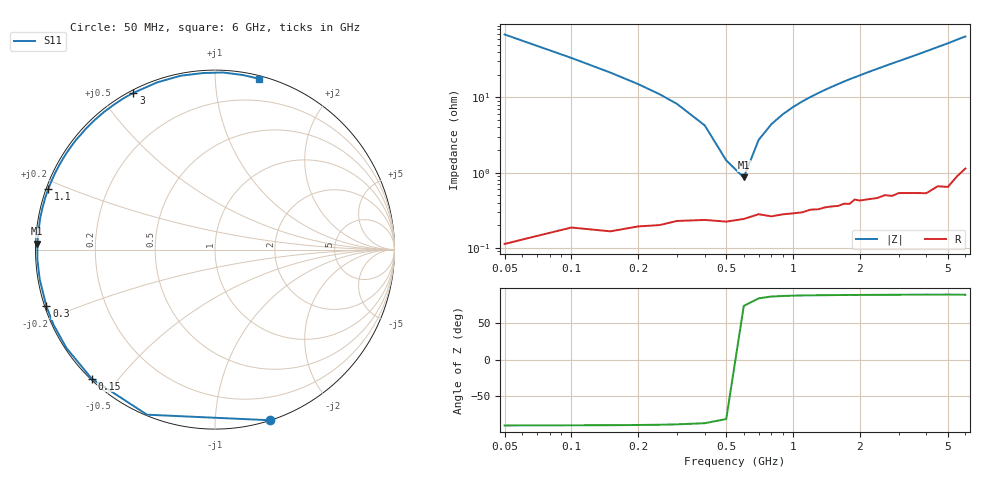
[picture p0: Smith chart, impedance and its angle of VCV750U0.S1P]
! Infineon Technologies  Discrete & RF Semiconductors
! BBY 56-03
! Si Tuning Diode in SOD323
! VR = 0.75 V
! S-Parameters:  June  1999
# GHz  S  MA  R  50
!  f  S11
! GHz  MAG  ANG
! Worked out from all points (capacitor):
!   34 points, 50 MHz to 6 GHz, reference 50 ohm
!   read as one part to ground: C = 46.1 pF near 50 MHz
!   lowest |Z| = 864 mohm at 600 MHz (marker M1)
!   series resonance near 563.5 MHz, so ESL is about 1.7 nH
!   S11 on the Smith chart (normalised r, x): 50 MHz: 0.00, -1.37; 150 MHz: 0.00, -0.43; 300 MHz: 0.00, -0.16; 1.1 GHz: 0.01, +0.18; 3 GHz: 0.01, +0.61; 6 GHz: 0.02, +1.29
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0.05  0.9984 -72.2
0.1  0.9949 -112.4
0.15  0.9944 -133.7
0.2  0.9929 -146.5
0.25  0.9923 -155.1
0.3  0.9911 -161.4
0.4  0.9907 -170.3
0.5  0.9911 -176.7
0.6  0.9903 178.1
0.7  0.9889 173.8
0.8  0.9896 169.9
1  0.9888 163.1
1.1  0.9885 160.0
1.3  0.9877 154.3
1.6  0.9868 146.5
1.8  0.9864 141.6
2  0.9853 137.2
2.2  0.9852 132.8
2.4  0.9851 128.8
2.6  0.9843 124.8
2.8  0.9852 121.1
3  0.9845 117.5
3.5  0.9858 109.1
4  0.9873 101.2
4.5  0.986 93.9
5  0.9877 87.4
5.5  0.985 81.0
6  0.9831 75.5
